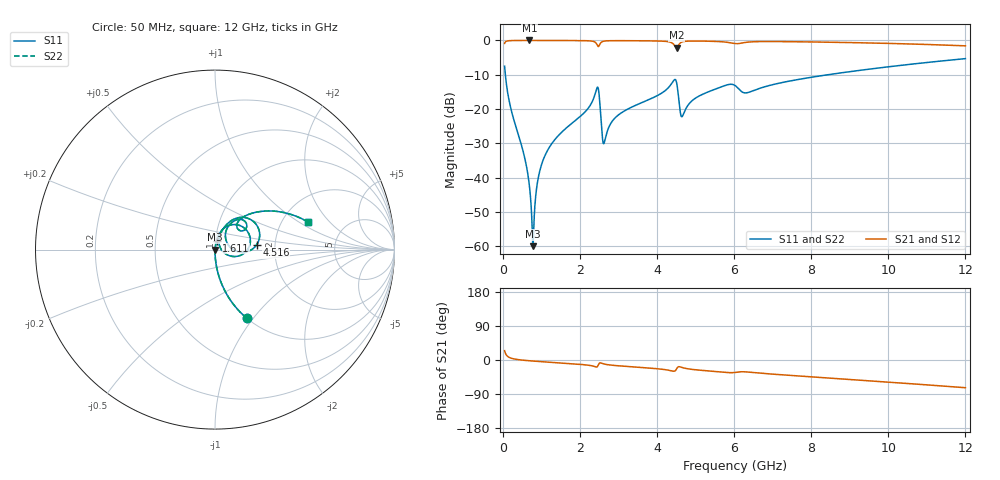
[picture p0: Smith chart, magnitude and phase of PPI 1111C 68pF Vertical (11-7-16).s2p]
# GHz S MA R 50
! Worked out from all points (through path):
!   1601 points, 50 MHz to 12 GHz, reference 50 ohm
!   highest |S21| = -0.01 dB at 692.3 MHz (marker M1); lowest = -2.1 dB at 4.509 GHz (marker M2)
!   group delay of S21, straight-line fit = 17 ps
!   lowest |S11| = -60.0 dB at 781.9 MHz (marker M3), VSWR 1.00, Z = 50.1 - j0.028 ohm
!   |S11| at or under -10 dB: 69.45 MHz to 8.441 GHz (8.371 GHz wide, 197 % of centre)
!   |S22| runs from -60.0 to -5.3 dB; largest |S21 - S12| = 0
!   S11 on the Smith chart (normalised r, x): 50 MHz: 1.00, -0.93; 1.611 GHz: 1.01, +0.10; 4.516 GHz: 1.60, +0.09; 12 GHz: 2.79, +1.20
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0.05  0.4211 -65.2  0.9067 24.7  0.9067 24.7  0.4211 -65.2
0.22925  0.09268 -85.1  0.9951 4.5  0.9951 4.5  0.09268 -85.1
0.557875  0.02083 -88.5  0.9989 -0.8  0.9989 -0.8  0.02083 -88.5
0.6923125  0.007616 -85.1  0.999 -2.0  0.999 -2.0  0.007616 -85.1
0.7819375  0.0009959 -16.3  0.999 -2.8  0.999 -2.8  0.0009959 -16.3
0.916375  0.009474 79.9  0.9989 -3.8  0.9989 -3.8  0.009474 79.9
1.035875  0.01717 81.6  0.9987 -4.7  0.9987 -4.7  0.01717 81.6
1.610969  0.05049 79.7  0.9971 -8.6  0.9971 -8.6  0.05049 79.7
2.044156  0.08081 76.0  0.9936 -11.9  0.9936 -11.9  0.08081 76.0
2.447469  0.204 35.3  0.8645 -18.1  0.8645 -18.1  0.204 35.3
2.641656  0.03336 42.2  0.9795 -10.9  0.9795 -10.9  0.03336 42.2
2.985219  0.08045 71.6  0.992 -15.1  0.992 -15.1  0.08045 71.6
4.038312  0.1597 64.3  0.9805 -23.4  0.9805 -23.4  0.1597 64.3
4.508844  0.2446 10.0  0.7867 -23.6  0.7867 -23.6  0.2446 10.0
4.516312  0.2335 6.5  0.7888 -22.3  0.7888 -22.3  0.2335 6.5
4.665687  0.07916 37.4  0.955 -20.2  0.955 -20.2  0.07916 37.4
5.083938  0.1534 60.1  0.979 -26.6  0.979 -26.6  0.1534 60.1
6.025  0.2201 36.4  0.9004 -32.9  0.9004 -32.9  0.2201 36.4
6.32375  0.1718 42.9  0.9397 -31.5  0.9397 -31.5  0.1718 42.9
8.019156  0.2909 44.3  0.9502 -44.5  0.9502 -44.5  0.2909 44.3
10.01331  0.4129 30.8  0.9049 -58.4  0.9049 -58.4  0.4129 30.8
12  0.5424 16.3  0.8337 -73.1  0.8337 -73.1  0.5424 16.3
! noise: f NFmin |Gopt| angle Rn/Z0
0.05  0.0004094  0.8776  0.4048  0.0007231
1.372  0.004162  0.7008  4.727  0.002719
2.701  0.01777  0.8504  9.504  0.02514
4.031  0.01563  0.7601  13.81  0.01302
5.36  0.02234  0.7764  18.37  0.01992
6.682  0.03299  0.8095  22.9  0.03468
8.012  0.02191  0.6844  26.29  0.01279
9.341  0.02235  0.652  29.73  0.01145
10.67  0.02445  0.6451  33.2  0.01203
12  0.02735  0.65  36.66  0.01344
